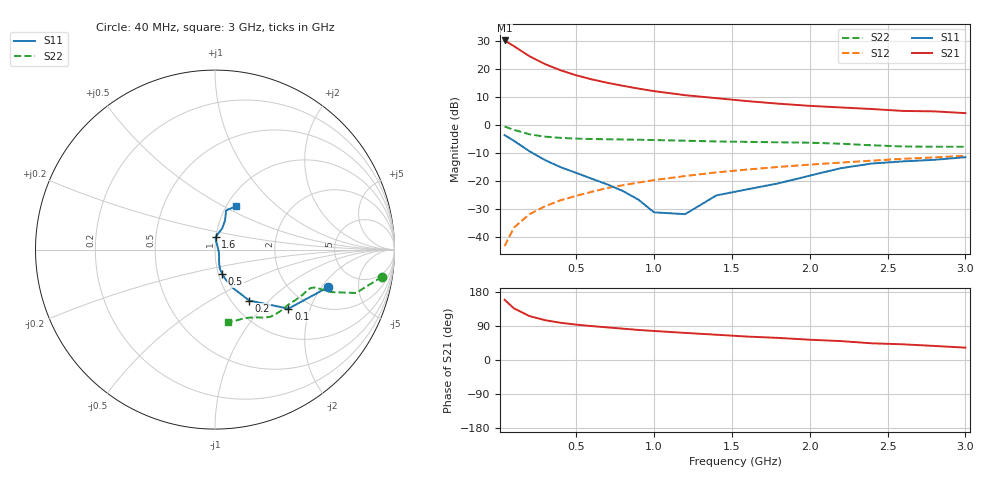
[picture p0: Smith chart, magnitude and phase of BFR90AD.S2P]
! Filename:  BFR90AD.S2P  Version:  2.0
! Philips part #: BFR90A  Date: Jul 1990
! Bias condition: Vce=5V, Ic=15mA
#  MHz  S  MA  R  50
! Freq  S11  S21  S12  S22  !GUM [dB]
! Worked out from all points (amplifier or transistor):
!   21 points, 40 MHz to 3 GHz, reference 50 ohm
!   highest |S21| = 30.1 dB at 40 MHz (marker M1)
!   |S21| within 3 dB of that: start of sweep to 126.8 MHz
!   unconditionally stable (mu >= 1): 523.2 MHz to end of sweep
!   at 300 MHz: K = 0.89, MSG = 25.3 dB, |S12| = -28.9 dB
!   at 1 GHz: K = 1.06, MAG = 14.3 dB, |S12| = -19.6 dB
!   at 3 GHz: K = 1.09, MAG = 5.7 dB, |S12| = -10.9 dB
!   S11 on the Smith chart (normalised r, x): 40 MHz: 3.09, -2.32; 100 MHz: 1.58, -1.44; 200 MHz: 1.20, -0.77; 500 MHz: 1.04, -0.29; 1.6 GHz: 1.00, +0.14; 3 GHz: 1.11, +0.58
40  0.664 -18.4  32.08 158.9  0.007 82.3  0.944 -9.2
100  0.525 -38.8  25.37 136.2  0.015 75.0  0.822 -17.1
200  0.342 -56.1  16.78 115.8  0.026 73.6  0.685 -20.2
300  0.238 -64.7  12.16 105.1  0.036 73.8  0.623 -20.5
400  0.178 -70.2  9.445 98.2  0.046 75.0  0.592 -20.9
500  0.141 -73.6  7.695 93.3  0.055 75.6  0.574 -21.9
600  0.111 -75.6  6.508 89.5  0.065 75.3  0.565 -23.1
700  0.088 -74.2  5.656 86.0  0.076 75.3  0.559 -24.5
800  0.067 -70.6  5.004 82.7  0.085 74.8  0.554 -26.0
900  0.047 -60.8  4.462 79.3  0.095 74.3  0.549 -27.4
1000  0.028 -38.4  4.021 76.6  0.105 73.7  0.542 -29.0
1200  0.026 59.7  3.404 71.5  0.124 72.1  0.527 -32.6
1400  0.056 86.0  3.016 66.7  0.144 70.7  0.511 -36.9
1600  0.072 86.1  2.668 61.8  0.162 69.1  0.503 -41.9
1800  0.092 78.3  2.404 58.3  0.18 67.8  0.494 -46.5
2000  0.126 71.3  2.2 53.5  0.198 66.0  0.486 -50.3
2200  0.171 71.0  2.06 49.9  0.215 64.1  0.466 -54.4
2400  0.207 73.1  1.931 44.0  0.233 62.6  0.437 -59.7
2600  0.226 74.3  1.786 41.4  0.251 60.3  0.416 -66.5
2800  0.241 70.3  1.755 37.1  0.266 58.9  0.412 -73.8
3000  0.268 63.9  1.633 32.6  0.284 57.9  0.411 -79.8
